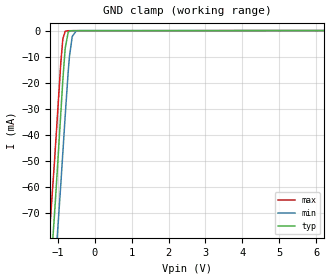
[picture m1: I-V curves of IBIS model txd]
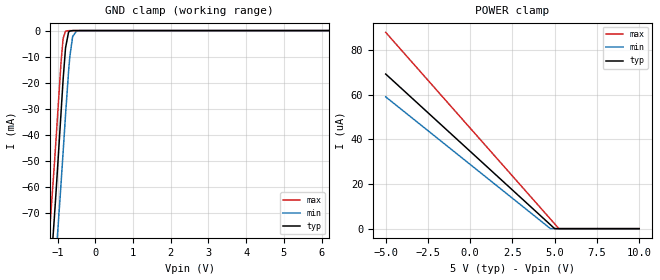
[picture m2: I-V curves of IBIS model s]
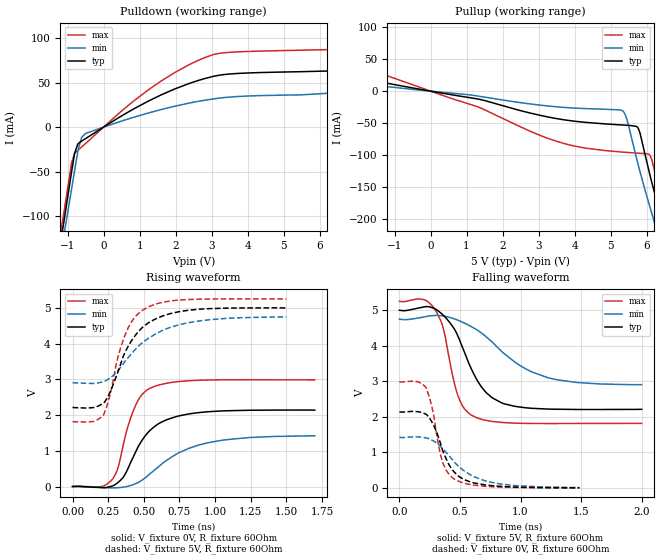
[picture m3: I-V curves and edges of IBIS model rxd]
|Texas Instruments Incorporated
|INDUSTRIAL CAN TRANSCEIVERS
|Marketing part#   Digital Voltage Range   Package-type   #pins
|SN65HVD252D   4.75V-5.25V   SOIC   8
|SN65HVD252DR   4.75V-5.25V   SOIC   8
[IBIS Ver]   4.1
[File name]   sn65hvd252.ibs
[File Rev]   1.0
[Date]   6/18/2016
[Source]
| Texas Instruments Incorporated.
| Analog-eLab Design Center, HPA
| 12500 TI Blvd
| Dallas, TX -75243
[Notes]   Revision History:
| Rev 1.0: 6/18/2016
| - Initial version of the model
| - Model generated from simulations in TISPICE
| - Model matched to SPICE simulation
| - C_comp although listed in numerical order of value are
|   obtained from varying PVT conditions. For PVT conditions for
|   each specific value refer the buffer description under
|   respective [Model]. IBIS model user is responsible for using
|   appropriate C_comp to simulate for Signal Integrity.
|* EXCEPTION:   *
|* - For s model there is leakage in power clamp due to resistor R2   *
|*   connected to pad.   *
|* - For txd model there is leakage in ground clamp due to resistor R2   *
|*   connected to pad.   *
|* - For canh_os,canl_od model there is leakage in power clamp and   *
|*   ground clamp tables due to resistor network connected to PAD.   *
[Disclaimer]
| This model is designed as an aid for customers of Texas Instruments.
| TI and its licensors and suppliers make no warranties, either expressed
| or implied, with respect to this  model, including the warranties of
| merchantability or fitness for a particular purpose. The model is
| provided solely on an "as is" basis. The entire risk as to its quality
| and performance is with the customer.
[Copyright]
(C) Copyright 2016 Texas Instruments Incorporated.All rights reserved.
|   SN65HVD252D
[Component]   SN65HVD252D
[Manufacturer]   TI
[Package]   |SOIC-8 - D Package
|   typ   min   max
R_pkg   0.077174   0.00230   0.11690
L_pkg   2.321345nH   1.36253nH   2.80112nH
C_pkg   0.398513pF   0.31326pF   0.46592pF
[Pin]  signal_name   model_name   R_pin   L_pin   C_pin
1   TXD   txd   0.11215   2.70023n   0.38408p
2   GND   gnd   0.03900   2.09764n   0.46592p
3   VCC   power   0.02513   1.85198n   0.46577p
4   RXD   rxd   0.11876   2.80112n   0.38992p
5   Vref   nc   0.00230   1.36253n   0.31326p
6   CANL   canl_od   0.11690   2.72346n   0.40067p
7   CANH   canh_os   0.09586   2.40528n   0.38694p
8   S   s   0.10729   2.62852n   0.38154p
[Diff_pin]   inv_pin   vdiff   tdelay_typ   tdelay_min   tdelay_max
7   6   NA   NA   NA   NA
| Models and submodels in the file (5): txd (Input), s (Input), rxd (Output), canh_os (Open_source), canl_od (Open_drain)
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|   txd Model
[Model]   txd
Model_type   Input
Vinl = 0.8
Vinh = 2
|   typ   min   max
|   (nom PVT)   (fast PVT)   (slow PVT)
C_comp   3.689e-13   3.534e-13   3.913e-13
| Where nom  PVT is Nominal Process, 5V, 27C
|   Fast PVT is Strong Process,  5.25V, -40C
|   Slow PVT is Weak Process,   4.75V, 125C
[Voltage Range]   5   4.75   5.25
|Ambient Temperature   25   85   -40
|Junction Temperature
[Temperature Range]   27   125   -40
[Power Clamp Reference]   5   4.75   5.25
[GND Clamp Reference]   0   0   0
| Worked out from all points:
|   GND clamp passes 1 mA (typ) near -0.72 V on its own axis
[GND Clamp]
|   Voltage   I(typ)   I(min)   I(max)
-5V       -570.9mA   -586.3mA   -524.8mA
-1.41V    -133.5mA   -153.2mA   -111.4mA
-1.204V   -95.06mA   -117mA     -74.28mA
-1.091V   -71.66mA   -95.34mA   -51.25mA
-1.045V   -61.68mA   -86.23mA   -41.34mA
-915.5mV  -31.84mA   -59.09mA   -12.47mA
-863mV    -19.73mA   -47.56mA   -3.695mA
-794.7mV  -6.64mA    -32.41mA   -269.8uA
-680mV    -194.6uA   -9.851mA   -53.14uA
-606.2mV  -37.88uA   -2.275mA   -51.66uA
-492.3mV  -27.95uA   -116.4uA   -51.51uA
10V       0A         0A         0A
[POWER Clamp]
|   Voltage   I(typ)   I(min)   I(max)
-5V       0A         0A         0A
0V        0A         0A         0A
10V       0A         0A         0A
|   s Model
[Model]   s
Model_type   Input
Vinl = 0.8
Vinh = 2.0
|   typ   min   max
|   (nom PVT)   (fast PVT)   (slow PVT)
C_comp   3.689e-13   3.534e-13   3.913e-13
| Where nom  PVT is Nominal Process, 5V, 27C
|   Fast PVT is Strong Process,  5.25V, -40C
|   Slow PVT is Weak Process,   4.75V, 125C
[Voltage Range]   5   4.75   5.25
|Ambient Temperature   25   85   -40
|Junction Temperature
[Temperature Range]   27   125   -40
[Power Clamp Reference]   5   4.75   5.25
[GND Clamp Reference]   0   0   0
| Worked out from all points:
|   GND clamp passes 1 mA (typ) near -0.72 V on its own axis
[GND Clamp]
|   Voltage   I(typ)   I(min)   I(max)
-5V       -570.9mA   -586.3mA   -524.8mA
-1.41V    -133.5mA   -153.2mA   -111.4mA
-1.204V   -95.05mA   -117mA     -74.26mA
-1.091V   -71.65mA   -95.34mA   -51.24mA
-1.045V   -61.67mA   -86.23mA   -41.32mA
-915.5mV  -31.84mA   -59.09mA   -12.45mA
-863mV    -19.72mA   -47.56mA   -3.675mA
-794.7mV  -6.632mA   -32.41mA   -247uA
-680mV    -178uA     -9.849mA   -20.22uA
-606.2mV  -16.59uA   -2.272mA   -11.03uA
-492.3mV  -3.718uA   -108.6uA   -4.74uA
10V       0A         0A         0A
[POWER Clamp]
|   Voltage   I(typ)   I(min)   I(max)
-5V       69.31uA    59.07uA    87.99uA
4.747V    1.753uA    18.18nA    4.317uA
4.995V    34.65nA    0A         2.189uA
5.248V    0A         0A         17.17nA
10V       0A         0A         0A
|   rxd Model
[Model]   rxd
Model_type   Output
Polarity   Non-Inverting
Vmeas = 2.5
Vref = 0
Cref = 15pF
Rref = 200
|   typ   min   max
|   (nom PVT)   (fast PVT)   (slow PVT)
C_comp   1.047e-12   9.672e-13   1.069e-12
| Where nom  PVT is Nominal Process, 5V, 27C
|   Fast PVT is Strong Process,  5.25V, -40C
|   Slow PVT is Weak Process,   4.75V, 125C
[Voltage Range]   5   4.75   5.25
|Ambient Temperature   25   85   -40
|Junction Temperature
[Temperature Range]   27   125   -40
[Pullup Reference]   5   4.75   5.25
[Pulldown Reference]   0   0   0
[Power Clamp Reference]   5   4.75   5.25
[GND Clamp Reference]   0   0   0
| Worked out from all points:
|   slope of the pulldown table from 0 to 0.75 V, typ, clamps not added: 40.7 ohm
|   slope of the pullup table from 0 to 0.75 V, typ, clamps not added: 104 ohm
|   falling waveform, V_fixture 5V, R_fixture 60Ohm: 20-80 % time 236ps typ, 419ps min, 138ps max; typ from 5 V to 2.21 V
|   rising waveform, V_fixture 0V, R_fixture 60Ohm: 20-80 % time 206ps typ, 343ps min, 133ps max; typ from 0 V to 2.14 V
|   rising waveform, V_fixture 5V, R_fixture 60Ohm: 20-80 % time 211ps typ, 314ps min, 148ps max; typ from 2.21 V to 5 V
|   falling waveform, V_fixture 0V, R_fixture 60Ohm: 20-80 % time 168ps typ, 287ps min, 112ps max; typ from 2.14 V to 0.001 V
[Pulldown]
|   Voltage   I(typ)   I(min)   I(max)
-5V       -902.4mA   -799.9mA   -1.017A
-1.167V   -121.9mA   -136.2mA   -111.6mA
-1.125V   -111.5mA   -126.5mA   -101.2mA
-891.2mV  -50.25mA   -69.74mA   -40.29mA
-801mV    -28.59mA   -47.21mA   -29.29mA
-695mV    -18.15mA   -23.04mA   -25.28mA
-500mV    -12.89mA   -7.141mA   -18.37mA
1.3V      30.31mA    16.44mA    43.42mA
2.82V     54.57mA    30.2mA     78.16mA
6.704V    63.4mA     39.12mA    87.34mA
8.48V     89.46mA    53.97mA    130.9mA
10V       117.3mA    69.15mA    177.2mA
[Pullup]
|   Voltage   I(typ)   I(min)   I(max)
-5V       57.41mA    34.8mA     98.23mA
1.303V    -12.23mA   -7.577mA   -24.42mA
3.32V     -41.19mA   -23.62mA   -75.29mA
5.274V    -52.92mA   -29.51mA   -95.33mA
5.441V    -53.46mA   -42.01mA   -96.05mA
5.77V     -58.4mA    -116mA     -97.34mA
6.098V    -132.4mA   -182.5mA   -100.9mA
6.214V    -157.8mA   -204.9mA   -123mA
6.366V    -188.8mA   -235.1mA   -158.7mA
6.524V    -218.9mA   -266.1mA   -191.8mA
6.635V    -240.8mA   -287.5mA   -213.3mA
10V       -901.7mA   -836.4mA   -962.5mA
[Ramp]
R_load = 60
|   typ   min   max
dV/dt_r   1.28313/2.05705e-10   0.852295/3.43359e-10   1.79127/1.32553e-10
dV/dt_f   1.67365/2.34995e-10   1.10683/4.18049e-10   2.06142/1.38024e-10
[Falling Waveform]
V_fixture = 5V
V_fixture_min = 4.75V
V_fixture_max = 5.25V
R_fixture = 60Ohm
|   Time   V(typ)   V(min)   V(max)
0s        5V         4.75V      5.25V
198ps     5.09V      4.808V     5.303V
300ps     5.028V     4.855V     4.984V
364ps     4.853V     4.838V     4.461V
482ps     4.28V      4.72V      2.609V
596ps     3.332V     4.534V     2.043V
760ps     2.55V      4.122V     1.872V
948ps     2.297V     3.555V     1.822V
1.304ns   2.213V     3.042V     1.811V
2ns       2.211V     2.905V     1.814V
[Rising Waveform]
V_fixture = 0V
V_fixture_min = 0V
V_fixture_max = 0V
R_fixture = 60Ohm
|   Time   V(typ)   V(min)   V(max)
0s        711.7pV    1.589nV    633.1pV
206ps     -32.05mV   -25.16mV   913.3uV
282ps     19.66mV    -37.63mV   213.9mV
318ps     108.7mV    -33.72mV   513.3mV
354ps     247.9mV    -19.46mV   1.131V
428ps     843.6mV    56.65mV    2.138V
544ps     1.574V     359.2mV    2.751V
734ps     1.964V     918.2mV    2.933V
946ps     2.092V     1.222V     2.981V
1.7ns     2.139V     1.42V      2.985V
[Rising Waveform]
V_fixture = 5V
V_fixture_min = 4.75V
V_fixture_max = 5.25V
R_fixture = 60Ohm
|   Time   V(typ)   V(min)   V(max)
0s        2.211V     2.905V     1.814V
150ps     2.213V     2.887V     1.824V
216ps     2.334V     2.938V     1.995V
268ps     2.684V     3.053V     2.655V
318ps     3.203V     3.245V     3.61V
368ps     3.755V     3.506V     4.236V
424ps     4.144V     3.765V     4.67V
496ps     4.473V     4.045V     4.946V
808ps     4.932V     4.583V     5.235V
1.5ns     5V         4.75V      5.25V
[Falling Waveform]
V_fixture = 0V
V_fixture_min = 0V
V_fixture_max = 0V
R_fixture = 60Ohm
|   Time   V(typ)   V(min)   V(max)
0s        2.139V     1.42V      2.985V
150ps     2.145V     1.435V     2.989V
216ps     2.077V     1.409V     2.839V
268ps     1.853V     1.344V     2.282V
324ps     1.405V     1.213V     1.176V
352ps     1.102V     1.121V     774.6mV
450ps     453.4mV    738.8mV    252.7mV
586ps     165.3mV    364.1mV    92.03mV
746ps     65.85mV    164.6mV    34.15mV
1.486ns   795uV      6.334mV    -576.6uV
